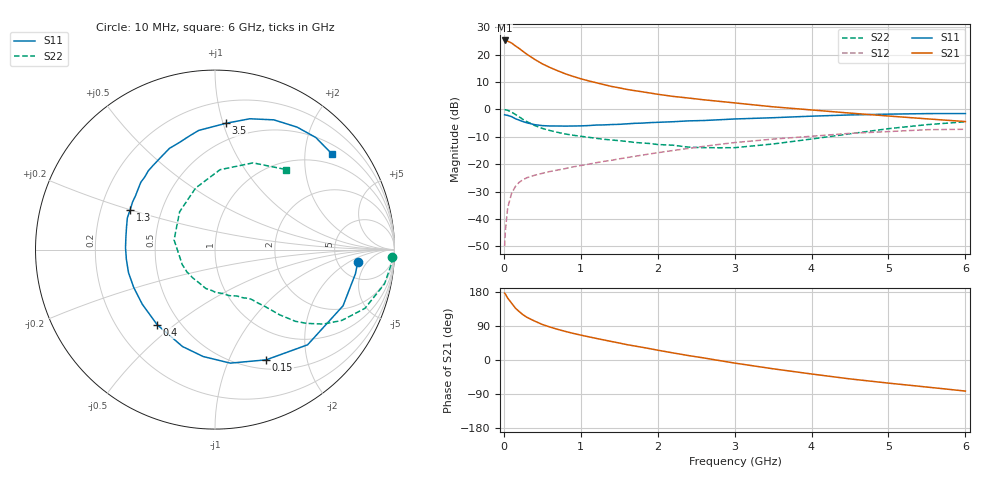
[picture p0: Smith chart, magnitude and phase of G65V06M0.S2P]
! SIEMENS Small Signal Semiconductors
! BFG193
! Si NPN RF Bipolar Junction Transistor in SOT223
! VCE = 5 V  IC = 6 mA
! Common Emitter S-Parameters:  August  1996
# GHz  S  MA  R  50
!  f  S11  S21  S12  S22
! GHz  MAG  ANG  MAG  ANG  MAG  ANG  MAG  ANG
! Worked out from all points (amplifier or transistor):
!   36 points, 10 MHz to 6 GHz, reference 50 ohm
!   highest |S21| = 25.2 dB at 10 MHz (marker M1)
!   |S21| within 3 dB of that: start of sweep to 203 MHz
!   unconditionally stable (mu >= 1): 1.05 GHz to 2.541 GHz
!   at 250 MHz: K = 0.38, MSG = 23.4 dB, |S12| = -25.6 dB
!   at 1.4 GHz: K = 1.08, MAG = 11.8 dB, |S12| = -18.6 dB
!   at 6 GHz: K = 0.87, MSG = 1.4 dB, |S12| = -7.2 dB
!   S11 on the Smith chart (normalised r, x): 10 MHz: 7.81, -2.95; 150 MHz: 0.61, -1.38; 400 MHz: 0.37, -0.44; 1.3 GHz: 0.33, +0.20; 3.5 GHz: 0.36, +1.02; 6 GHz: 0.71, +2.62
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0.01  0.7988 -4.9  18.15 176.5  0.0032 88.9  0.9882 -2.4
0.02  0.7938 -9.8  18.01 174.1  0.0061 85.7  0.9863 -4.6
0.05  0.7791 -23.7  17.62 163.3  0.0161 76.8  0.9638 -11.4
0.1  0.7399 -45.8  16.32 150.2  0.0292 68.9  0.8973 -21.4
0.15  0.6771 -65.1  14.47 137.0  0.0393 59.4  0.809 -29.2
0.2  0.6383 -82.3  12.95 127.7  0.0469 54.1  0.7326 -34.5
0.25  0.5994 -96.3  11.45 119.3  0.0524 49.6  0.6561 -38.8
0.3  0.5697 -108.5  10.16 112.7  0.0568 47.5  0.6008 -41.7
0.4  0.5282 -127.6  8.219 102.7  0.0629 43.9  0.5105 -45.3
0.5  0.5068 -143.1  6.795 93.8  0.0682 42.2  0.4509 -47.4
0.6  0.4995 -155.0  5.827 87.0  0.0738 42.0  0.412 -49.2
0.7  0.4988 -165.0  5.079 80.9  0.0784 42.1  0.3821 -51.2
0.9  0.4986 178.8  4.012 70.3  0.0896 42.2  0.3384 -54.3
1.1  0.508 166.1  3.327 61.3  0.1001 42.8  0.3104 -59.8
1.3  0.5221 155.2  2.842 52.9  0.1129 42.5  0.2854 -64.8
1.6  0.5466 141.3  2.32 40.5  0.1324 40.8  0.2605 -75.6
2.2  0.597 120.2  1.731 18.7  0.1783 34.4  0.2226 -103.3
2.8  0.6485 102.8  1.405 -1.4  0.2308 24.6  0.1999 -141.6
3.5  0.7066 85.0  1.117 -23.2  0.2878 9.7  0.2343 166.7
4.5  0.7938 65.6  0.858 -49.9  0.3664 -10.7  0.3595 107.5
5.5  0.8398 48.1  0.674 -71.4  0.4273 -36.3  0.5278 66.3
6  0.8418 39.4  0.601 -82.0  0.4347 -51.0  0.5957 48.5
